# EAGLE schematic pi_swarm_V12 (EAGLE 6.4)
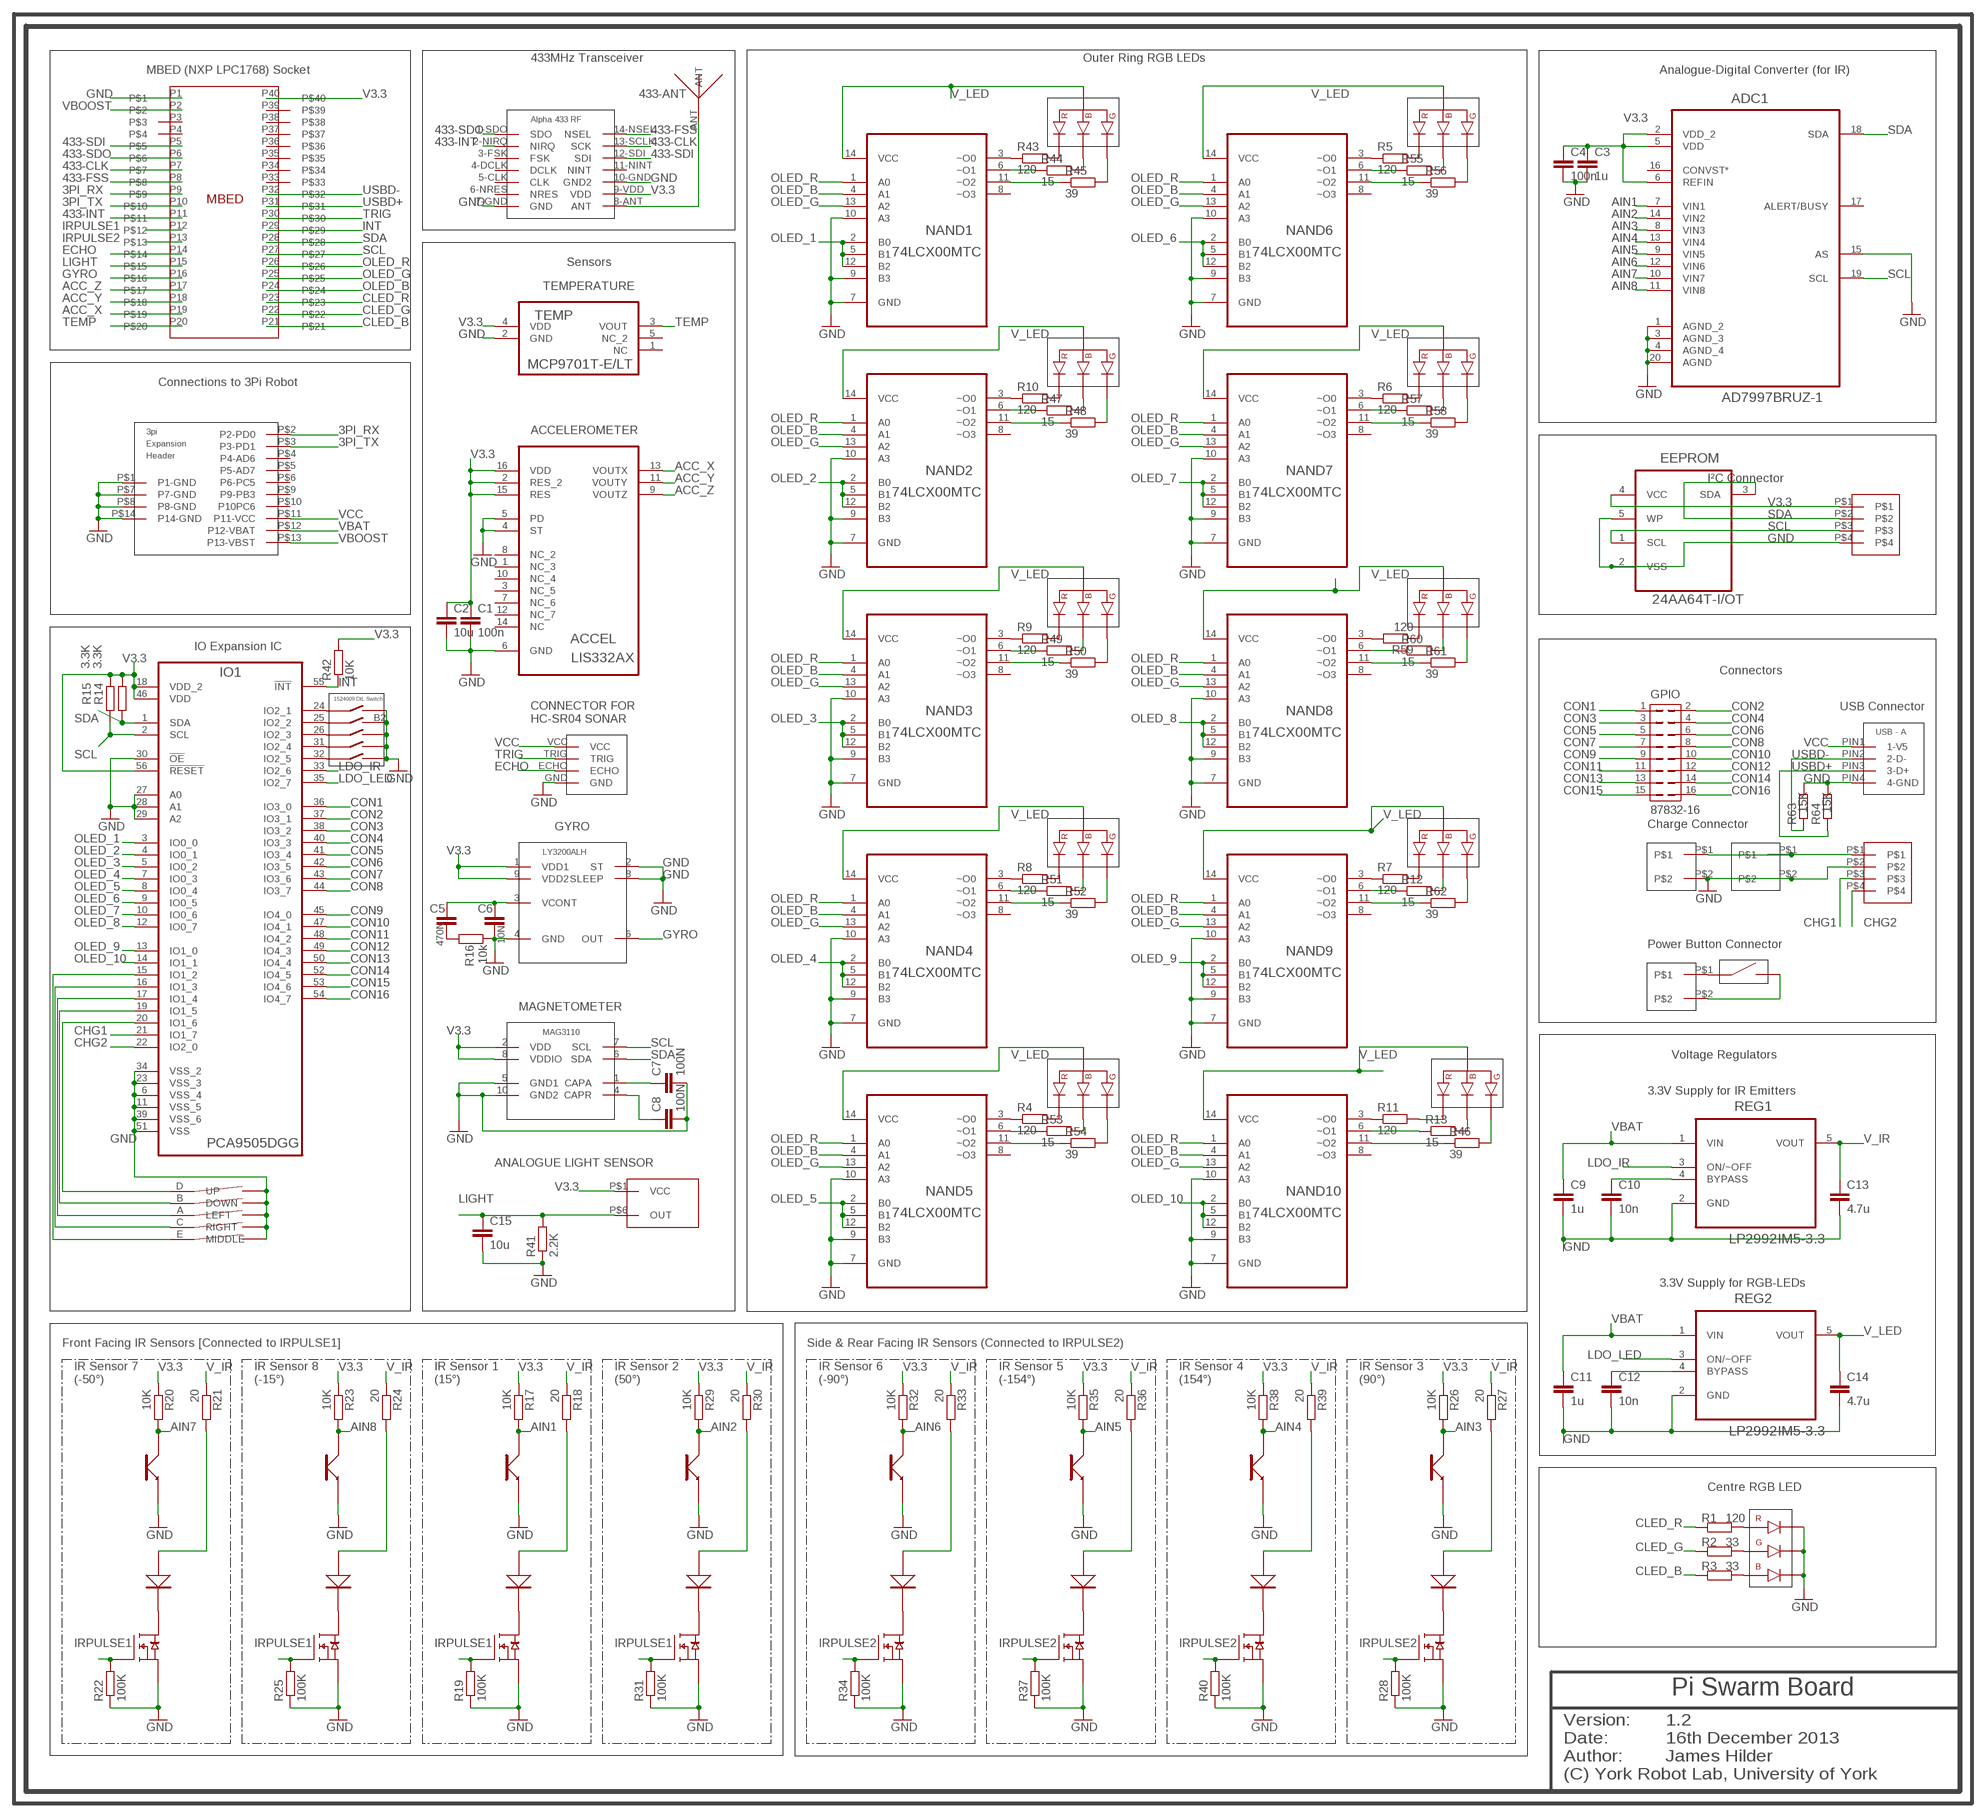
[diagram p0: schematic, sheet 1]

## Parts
3PI_HEADER  3PI-EXPANSION-HEADER  [9689605-2X7-SM-HEADER]
ACCEL  LIS332AX  [LGA16R50P3X5_300X300X100]
ADC1  AD7997BRUZ-1  [SOP65P640X120-20N]
ALPHA433  ALPHA433  [ALPHA433]
ANTENNA  ANTENNA  [2148530-433MHZANTENNA]
C1  100n  C-EUC0603  [C0603]
C2  10u  C-EUC0603  [C0603]
C3  1u  C-EUC0603  [C0603]
C4  100n  C-EUC0603  [C0603]
C5  470N  C-EUC0603  [C0603]
C6  10N  C-EUC0603  [C0603]
C7  100N  C-EUC0603  [C0603]
C8  100N  C-EUC0603  [C0603]
C9  1u  C-EUC0805K  [C0805K]
C10  10n  C-EUC0805K  [C0805K]
C11  1u  C-EUC0805K  [C0805K]
C12  10n  C-EUC0805K  [C0805K]
C13  4.7u  C-EUC1206K  [C1206K]
C14  4.7u  C-EUC1206K  [C1206K]
C15  10u  C-EUC0603K  [C0603K]
CENTRE_LED  CREE-CLP6C-FKG-RGBLED  [CREE-CLP6C-RGB-LED]
CHG_IN  2-PIN-CONNECTOR  [2-PIN-CONNECTOR]
CHG_OUT  2-PIN-CONNECTOR  [2-PIN-CONNECTOR]
EEPROM  24AA64T-I/OT  [SOT95P270X145-5N]
GPIO  87832-16  [87832-16]
GYRO  GYRO-LY3200ALH-1838547  [GYRO-1838547]
I2C_CONN  4-PIN-CONNECTOR-9492437  [4PIN-2MM-CON]
IO1  PCA9505DGG  [SOP50P810X120-56N]
IR1  TCRT1000-IR  [TCRT1000-IR]
IR2  TCRT1000-IR  [TCRT1000-IR]
IR3  TCRT1000-IR  [TCRT1000-IR]
IR4  TCRT1000-IR  [TCRT1000-IR]
IR5  TCRT1000-IR  [TCRT1000-IR]
IR6  TCRT1000-IR  [TCRT1000-IR]
IR7  TCRT1000-IR  [TCRT1000-IR]
IR8  TCRT1000-IR  [TCRT1000-IR]
LED1  KINGBRIGHT-RGL-RA-LED-2335788  [KINGBRIGHT-RA-RGB-LED]
LED2  KINGBRIGHT-RGL-RA-LED-2335788  [KINGBRIGHT-RA-RGB-LED]
LED3  KINGBRIGHT-RGL-RA-LED-2335788  [KINGBRIGHT-RA-RGB-LED]
LED4  KINGBRIGHT-RGL-RA-LED-2335788  [KINGBRIGHT-RA-RGB-LED]
LED5  KINGBRIGHT-RGL-RA-LED-2335788  [KINGBRIGHT-RA-RGB-LED]
LED6  KINGBRIGHT-RGL-RA-LED-2335788  [KINGBRIGHT-RA-RGB-LED]
LED7  KINGBRIGHT-RGL-RA-LED-2335788  [KINGBRIGHT-RA-RGB-LED]
LED8  KINGBRIGHT-RGL-RA-LED-2335788  [KINGBRIGHT-RA-RGB-LED]
LED9  KINGBRIGHT-RGL-RA-LED-2335788  [KINGBRIGHT-RA-RGB-LED]
LED10  KINGBRIGHT-RGL-RA-LED-2335788  [KINGBRIGHT-RA-RGB-LED]
LIGHTSENSOR  APDS-9005-020LIGHTSENSOR-1548110  [APDS-9005-020-LIGHTSENSOR-1548110]
MAGNETO  MAG3310-MAGNETOMETER-2080492  [MAG3110]
MBED  MBED  [MBED40PINDIL]
N1  IRLML2402-NMOS  [SOT23]
N2  IRLML2402-NMOS  [SOT23]
N3  IRLML2402-NMOS  [SOT23]
N4  IRLML2402-NMOS  [SOT23]
N5  IRLML2402-NMOS  [SOT23]
N6  IRLML2402-NMOS  [SOT23]
N7  IRLML2402-NMOS  [SOT23]
N8  IRLML2402-NMOS  [SOT23]
NAND1  74LCX00MTC  [SOP65P640X120-14N]
NAND2  74LCX00MTC  [SOP65P640X120-14N]
NAND3  74LCX00MTC  [SOP65P640X120-14N]
NAND4  74LCX00MTC  [SOP65P640X120-14N]
NAND5  74LCX00MTC  [SOP65P640X120-14N]
NAND6  74LCX00MTC  [SOP65P640X120-14N]
NAND7  74LCX00MTC  [SOP65P640X120-14N]
NAND8  74LCX00MTC  [SOP65P640X120-14N]
NAND9  74LCX00MTC  [SOP65P640X120-14N]
NAND10  74LCX00MTC  [SOP65P640X120-14N]
POWER_CON  2-PIN-CONNECTOR  [2-PIN-CONNECTOR]
R1  120  R-EU_R0603  [R0603]
R2  33  R-EU_R0603  [R0603]
R3  33  R-EU_R0603  [R0603]
R4  120  R-EU_R0603  [R0603]
R5  120  R-EU_R0603  [R0603]
R6  120  R-EU_R0603  [R0603]
R7  120  R-EU_R0603  [R0603]
R8  120  R-EU_R0603  [R0603]
R9  120  R-EU_R0603  [R0603]
R10  120  R-EU_R0603  [R0603]
R11  120  R-EU_R0603  [R0603]
R12  15  R-EU_R0603  [R0603]
R13  15  R-EU_R0603  [R0603]
R14  3.3K  R-EU_R0603  [R0603]
R15  3.3K  R-EU_R0603  [R0603]
R16  10k  R-EU_R0603  [R0603]
R17  10K  R-EU_R0603  [R0603]
R18  20  R-EU_R0603  [R0603]
R19  100K  R-EU_R0603  [R0603]
R20  10K  R-EU_R0603  [R0603]
R21  20  R-EU_R0603  [R0603]
R22  100K  R-EU_R0603  [R0603]
R23  10K  R-EU_R0603  [R0603]
R24  20  R-EU_R0603  [R0603]
R25  100K  R-EU_R0603  [R0603]
R26  10K  R-EU_R0603  [R0603]
R27  20  R-EU_R0603  [R0603]
R28  100K  R-EU_R0603  [R0603]
R29  10K  R-EU_R0603  [R0603]
R30  20  R-EU_R0603  [R0603]
R31  100K  R-EU_R0603  [R0603]
R32  10K  R-EU_R0603  [R0603]
R33  20  R-EU_R0603  [R0603]
R34  100K  R-EU_R0603  [R0603]
R35  10K  R-EU_R0603  [R0603]
R36  20  R-EU_R0603  [R0603]
R37  100K  R-EU_R0603  [R0603]
R38  10K  R-EU_R0603  [R0603]
R39  20  R-EU_R0603  [R0603]
R40  100K  R-EU_R0603  [R0603]
R41  2.2K  R-EU_R0603  [R0603]
R42  10K  R-EU_R0603  [R0603]
R43  120  R-EU_R0603  [R0603]
R44  15  R-EU_R0603  [R0603]
R45  39  R-EU_R0603  [R0603]
R46  39  R-EU_R0603  [R0603]
R47  15  R-EU_R0603  [R0603]
R48  39  R-EU_R0603  [R0603]
R49  15  R-EU_R0603  [R0603]
R50  39  R-EU_R0603  [R0603]
R51  15  R-EU_R0603  [R0603]
R52  39  R-EU_R0603  [R0603]
R53  15  R-EU_R0603  [R0603]
R54  39  R-EU_R0603  [R0603]
R55  15  R-EU_R0603  [R0603]
R56  39  R-EU_R0603  [R0603]
R57  15  R-EU_R0603  [R0603]
R58  39  R-EU_R0603  [R0603]
R59  120  R-EU_R0603  [R0603]
R60  15  R-EU_R0603  [R0603]
R61  39  R-EU_R0603  [R0603]
R62  39  R-EU_R0603  [R0603]
R63  15K  R-EU_R0402  [R0402]
R64  15K  R-EU_R0402  [R0402]
REG1  LP2992IM5-3.3  [SOT95P284X122-5N]
REG2  LP2992IM5-3.3  [SOT95P284X122-5N]
SONAR_CON  4-PIN-CONNECTOR-2084263  [4-PIN-CONNECTOR-2084263]
SWITCH1  1703878-SWITCH  [SWITCH-1703878]
SWITCH2  5WAYSWITCH-MCTT5V-1316988  [5WAYSWITCH]
SWITCH3  5PINDIPSWITCH-1524009  [5DIPSWITCH-1524009]
TEMP  MCP9701T-E/LT  [SOT65P210X110-5N]
U$1  4PIN-CON-177295  [4-PIN-CONNECTOR-1772951]
USB_CONNECTOR  USB-1654064  [USB-A-1654064]

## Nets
3PI_RX: 3PI_HEADER.P$2(P2-PD0) MBED.P9
3PI_TX: 3PI_HEADER.P$3(P3-PD1) MBED.P10
433-ANT: ALPHA433.8-ANT(ANT) ANTENNA.ANT
433-CLK: ALPHA433.13-SCLK(SCK) MBED.P7
433-FSS: ALPHA433.14-NSEL(NSEL) MBED.P8
433-INT: ALPHA433.2-NIRQ(NIRQ) MBED.P11
433-SDI: ALPHA433.12-SDI(SDI) MBED.P5
433-SDO: ALPHA433.1-SDO(SDO) MBED.P6
ACC_X: ACCEL.13(VOUTX) MBED.P19
ACC_Y: ACCEL.11(VOUTY) MBED.P18
ACC_Z: ACCEL.9(VOUTZ) MBED.P17
AIN1: ADC1.7(VIN1) IR1.4-COLLECTOR(CO) R17.2
AIN2: ADC1.14(VIN2) IR2.4-COLLECTOR(CO) R29.2
AIN3: ADC1.8(VIN3) IR3.4-COLLECTOR(CO) R26.2
AIN4: ADC1.13(VIN4) IR4.4-COLLECTOR(CO) R38.2
AIN5: ADC1.9(VIN5) IR5.4-COLLECTOR(CO) R35.2
AIN6: ADC1.12(VIN6) IR6.4-COLLECTOR(CO) R32.2
AIN7: ADC1.10(VIN7) IR7.4-COLLECTOR(CO) R20.2
AIN8: ADC1.11(VIN8) IR8.4-COLLECTOR(CO) R23.2
CHG1: IO1.21(IO1_7) U$1.P$3
CHG2: IO1.22(IO2_0) U$1.P$4
CLED_B: MBED.P21 R3.1
CLED_G: MBED.P22 R2.1
CLED_R: MBED.P23 R1.1
CON1: GPIO.1 IO1.36(IO3_0)
CON2: GPIO.2 IO1.37(IO3_1)
CON3: GPIO.3 IO1.38(IO3_2)
CON4: GPIO.4 IO1.40(IO3_3)
CON5: GPIO.5 IO1.41(IO3_4)
CON6: GPIO.6 IO1.42(IO3_5)
CON7: GPIO.7 IO1.43(IO3_6)
CON8: GPIO.8 IO1.44(IO3_7)
CON9: GPIO.9 IO1.45(IO4_0)
CON10: GPIO.10 IO1.47(IO4_1)
CON11: GPIO.11 IO1.48(IO4_2)
CON12: GPIO.12 IO1.49(IO4_3)
CON13: GPIO.13 IO1.50(IO4_4)
CON14: GPIO.14 IO1.52(IO4_5)
CON15: GPIO.15 IO1.53(IO4_6)
CON16: GPIO.16 IO1.54(IO4_7)
ECHO: MBED.P14 SONAR_CON.ECHO
GND: 3PI_HEADER.P$1(P1-GND) 3PI_HEADER.P$7(P7-GND) 3PI_HEADER.P$8(P8-GND) 3PI_HEADER.P$14(P14-GND) ACCEL.4(ST) ACCEL.5(PD) ACCEL.6(GND) ADC1.1(AGND_2) ADC1.3(AGND_3) ADC1.4(AGND_4) ADC1.15(AS) ADC1.20(AGND) ALPHA433.7-GND(GND) ALPHA433.10-GND(GND2) C1.2 C2.2 C3.2 C4.2 C6.2 C7.2 C8.2 C9.2 C10.2 C11.2 C12.2 C13.2 C14.2 C15.2 CENTRE_LED.P$4 CENTRE_LED.P$5 CENTRE_LED.P$6 CHG_IN.P$2 CHG_OUT.P$2 EEPROM.2(VSS) EEPROM.5(WP) GYRO.2(ST) GYRO.4(GND) GYRO.8(SLEEP) I2C_CONN.P$4 IO1.6(VSS_4) IO1.11(VSS_5) IO1.23(VSS_3) IO1.27(A0) IO1.28(A1) IO1.29(A2) IO1.30(!OE) IO1.34(VSS_2) IO1.39(VSS_6) IO1.51(VSS) IR1.3-EMITTER(EM) IR2.3-EMITTER(EM) IR3.3-EMITTER(EM) IR4.3-EMITTER(EM) IR5.3-EMITTER(EM) IR6.3-EMITTER(EM) IR7.3-EMITTER(EM) IR8.3-EMITTER(EM) MAGNETO.5(GND1) MAGNETO.10(GND2) MBED.P1 N1.2(2:S) N2.2(2:S) N3.2(2:S) N4.2(2:S) N5.2(2:S) N6.2(2:S) N7.2(2:S) N8.2(2:S) NAND1.7(GND) NAND1.9(B3) NAND1.10(A3) NAND2.7(GND) NAND2.9(B3) NAND2.10(A3) NAND3.7(GND) NAND3.9(B3) NAND3.10(A3) NAND4.7(GND) NAND4.9(B3) NAND4.10(A3) NAND5.7(GND) NAND5.9(B3) NAND5.10(A3) NAND6.7(GND) NAND6.9(B3) NAND6.10(A3) NAND7.7(GND) NAND7.9(B3) NAND7.10(A3) NAND8.7(GND) NAND8.9(B3) NAND8.10(A3) NAND9.7(GND) NAND9.9(B3) NAND9.10(A3) NAND10.7(GND) NAND10.9(B3) NAND10.10(A3) R16.1 R19.1 R22.1 R25.1 R28.1 R31.1 R34.1 R37.1 R40.1 R41.1 R63.2 R64.2 REG1.2(GND) REG2.2(GND) SONAR_CON.GND SWITCH2.COM1(LEFT_COMMON) SWITCH2.COM2(DOWN_COMMON) SWITCH2.COM3(UP_COMMON) SWITCH2.COM4(RIGHT_COMMON) SWITCH2.COM5(MIDDLE_COMMON) SWITCH3.A2 SWITCH3.B2 SWITCH3.C2 SWITCH3.D2 SWITCH3.E2 TEMP.2(GND) U$1.P$2 USB_CONNECTOR.PIN4(4-GND)
GYRO: GYRO.6(OUT) MBED.P16
INT: IO1.55(!INT) MBED.P29 R42.1
IRPULSE1: MBED.P12 N1.1(1:G) N2.1(1:G) N7.1(1:G) N8.1(1:G) R19.2 R22.2 R25.2 R31.2
IRPULSE2: MBED.P13 N3.1(1:G) N4.1(1:G) N5.1(1:G) N6.1(1:G) R28.2 R34.2 R37.2 R40.2
LDO_IR: IO1.33(IO2_6) REG1.3(ON/~OFF)
LDO_LED: IO1.35(IO2_7) REG2.3(ON/~OFF)
LIGHT: C15.1 LIGHTSENSOR.P$6(OUT) MBED.P15 R41.2
N$1: CENTRE_LED.P$1 R1.2
N$2: CENTRE_LED.P$2 R2.2
N$3: CENTRE_LED.P$3 R3.2
N$4: POWER_CON.P$1 SWITCH1.1
N$5: POWER_CON.P$2 SWITCH1.2
N$6: LED5.PIN1(RED_CATHODE) R4.2
N$7: LED6.PIN1(RED_CATHODE) R5.2
N$8: LED7.PIN1(RED_CATHODE) R6.2
N$9: NAND9.3(~O0) R7.1
N$10: LED4.PIN1(RED_CATHODE) R8.2
N$11: LED3.PIN1(RED_CATHODE) R9.2
N$12: LED2.PIN1(RED_CATHODE) R10.2
N$13: NAND10.3(~O0) R11.1
N$14: LED9.PIN4(BLUE_CATHODE) R12.2
N$15: LED10.PIN1(RED_CATHODE) R11.2
N$16: LED1.PIN1(RED_CATHODE) R43.2
N$17: NAND1.6(~O1) R44.1
N$18: LED1.PIN4(BLUE_CATHODE) R44.2
N$19: NAND2.3(~O0) R10.1
N$20: LED2.PIN4(BLUE_CATHODE) R47.2
N$21: LED2.PIN3(GREEN_CATHODE) R48.2
N$22: NAND3.3(~O0) R9.1
N$23: NAND3.6(~O1) R49.1
N$24: LED3.PIN4(BLUE_CATHODE) R49.2
N$25: NAND4.3(~O0) R8.1
N$26: NAND4.6(~O1) R51.1
N$27: NAND4.11(~O2) R52.1
N$28: NAND5.3(~O0) R4.1
N$29: NAND5.6(~O1) R53.1
N$30: NAND5.11(~O2) R54.1
N$31: NAND6.3(~O0) R5.1
N$32: NAND6.6(~O1) R55.1
N$33: NAND6.11(~O2) R56.1
N$34: NAND7.3(~O0) R6.1
N$35: LED7.PIN4(BLUE_CATHODE) R57.2
N$36: LED7.PIN3(GREEN_CATHODE) R58.2
N$37: NAND8.3(~O0) R59.2
N$38: NAND8.6(~O1) R60.1
N$39: LED8.PIN3(GREEN_CATHODE) R61.2
N$40: LED9.PIN1(RED_CATHODE) R7.2
N$41: NAND9.6(~O1) R12.1
N$42: NAND9.11(~O2) R62.1
N$43: LED10.PIN4(BLUE_CATHODE) R13.2
N$44: NAND10.6(~O1) R13.1
N$45: NAND10.11(~O2) R46.1
N$46: CHG_IN.P$1 CHG_OUT.P$1 U$1.P$1
N$47: C5.2 R16.2
N$48: C7.1 MAGNETO.1(CAPA)
N$49: C5.1 C6.1 GYRO.3(VCONT)
N$50: C8.1 MAGNETO.4(CAPR)
N$51: IR1.2-CATHODE(CA) N1.3(3:D)
N$52: C12.1 REG2.4(BYPASS)
N$53: C10.1 REG1.4(BYPASS)
N$54: IR7.2-CATHODE(CA) N7.3(3:D)
N$55: IR7.1-ANODE(AN) R21.2
N$56: IR1.1-ANODE(AN) R18.2
N$57: IR8.1-ANODE(AN) R24.2
N$58: IR8.2-CATHODE(CA) N8.3(3:D)
N$59: IR3.1-ANODE(AN) R27.2
N$60: IR3.2-CATHODE(CA) N3.3(3:D)
N$61: IR2.1-ANODE(AN) R30.2
N$62: IO1.15(IO1_2) SWITCH2.E(MIDDLE)
N$63: IO1.16(IO1_3) SWITCH2.C(RIGHT)
N$64: IO1.17(IO1_4) SWITCH2.A(LEFT)
N$65: IO1.19(IO1_5) SWITCH2.B(DOWN)
N$66: IO1.20(IO1_6) SWITCH2.D(UP)
N$67: IO1.24(IO2_1) SWITCH3.A1
N$68: IO1.25(IO2_2) SWITCH3.B1
N$69: IO1.26(IO2_3) SWITCH3.C1
N$70: IO1.31(IO2_4) SWITCH3.D1
N$71: IO1.32(IO2_5) SWITCH3.E1
N$72: IR6.1-ANODE(AN) R33.2
N$73: IR2.2-CATHODE(CA) N2.3(3:D)
N$74: IR5.1-ANODE(AN) R36.2
N$75: IR6.2-CATHODE(CA) N6.3(3:D)
N$76: IR5.2-CATHODE(CA) N5.3(3:D)
N$77: IR4.1-ANODE(AN) R39.2
N$78: IR4.2-CATHODE(CA) N4.3(3:D)
N$79: NAND1.3(~O0) R43.1
N$80: LED1.PIN3(GREEN_CATHODE) R45.2
N$81: NAND1.11(~O2) R45.1
N$82: LED10.PIN3(GREEN_CATHODE) R46.2
N$83: NAND2.6(~O1) R47.1
N$84: NAND2.11(~O2) R48.1
N$85: LED3.PIN3(GREEN_CATHODE) R50.2
N$86: NAND3.11(~O2) R50.1
N$87: LED4.PIN3(GREEN_CATHODE) R52.2
N$88: LED4.PIN4(BLUE_CATHODE) R51.2
N$89: LED5.PIN3(GREEN_CATHODE) R54.2
N$90: LED5.PIN4(BLUE_CATHODE) R53.2
N$91: LED6.PIN4(BLUE_CATHODE) R55.2
N$92: LED6.PIN3(GREEN_CATHODE) R56.2
N$93: NAND7.6(~O1) R57.1
N$94: NAND7.11(~O2) R58.1
N$95: LED8.PIN1(RED_CATHODE) R59.1
N$96: LED8.PIN4(BLUE_CATHODE) R60.2
N$97: NAND8.11(~O2) R61.1
N$98: LED9.PIN3(GREEN_CATHODE) R62.2
OLED_1: IO1.3(IO0_0) NAND1.2(B0) NAND1.5(B1) NAND1.12(B2)
OLED_2: IO1.4(IO0_1) NAND2.2(B0) NAND2.5(B1) NAND2.12(B2)
OLED_3: IO1.5(IO0_2) NAND3.2(B0) NAND3.5(B1) NAND3.12(B2)
OLED_4: IO1.7(IO0_3) NAND4.2(B0) NAND4.5(B1) NAND4.12(B2)
OLED_5: IO1.8(IO0_4) NAND5.2(B0) NAND5.5(B1) NAND5.12(B2)
OLED_6: IO1.9(IO0_5) NAND6.2(B0) NAND6.5(B1) NAND6.12(B2)
OLED_7: IO1.10(IO0_6) NAND7.2(B0) NAND7.5(B1) NAND7.12(B2)
OLED_8: IO1.12(IO0_7) NAND8.2(B0) NAND8.5(B1) NAND8.12(B2)
OLED_9: IO1.13(IO1_0) NAND9.2(B0) NAND9.5(B1) NAND9.12(B2)
OLED_10: IO1.14(IO1_1) NAND10.2(B0) NAND10.5(B1) NAND10.12(B2)
OLED_B: MBED.P24 NAND1.4(A1) NAND2.4(A1) NAND3.4(A1) NAND4.4(A1) NAND5.4(A1) NAND6.4(A1) NAND7.4(A1) NAND8.4(A1) NAND9.4(A1) NAND10.4(A1)
OLED_G: MBED.P25 NAND1.13(A2) NAND2.13(A2) NAND3.13(A2) NAND4.13(A2) NAND5.13(A2) NAND6.13(A2) NAND7.13(A2) NAND8.13(A2) NAND9.13(A2) NAND10.13(A2)
OLED_R: MBED.P26 NAND1.1(A0) NAND2.1(A0) NAND3.1(A0) NAND4.1(A0) NAND5.1(A0) NAND6.1(A0) NAND7.1(A0) NAND8.1(A0) NAND9.1(A0) NAND10.1(A0)
SCL: ADC1.19(SCL) EEPROM.1(SCL) I2C_CONN.P$3 IO1.2(SCL) MAGNETO.7(SCL) MBED.P27 R15.1
SDA: ADC1.18(SDA) EEPROM.3(SDA) I2C_CONN.P$2 IO1.1(SDA) MAGNETO.6(SDA) MBED.P28 R14.1
TEMP: MBED.P20 TEMP.3(VOUT)
TRIG: MBED.P30 SONAR_CON.TRIG
USBD+: MBED.P31 R64.1 USB_CONNECTOR.PIN3(3-D+)
USBD-: MBED.P32 R63.1 USB_CONNECTOR.PIN2(2-D-)
V3.3: ACCEL.2(RES_2) ACCEL.15(RES) ACCEL.16(VDD) ADC1.2(VDD_2) ADC1.5(VDD) ADC1.6(REFIN) ALPHA433.9-VDD(VDD) C1.1 C2.1 C3.1 C4.1 EEPROM.4(VCC) GYRO.1(VDD1) GYRO.9(VDD2) I2C_CONN.P$1 IO1.18(VDD_2) IO1.46(VDD) IO1.56(!RESET) LIGHTSENSOR.P$1(VCC) MAGNETO.2(VDD) MAGNETO.8(VDDIO) MBED.P40 R14.2 R15.2 R17.1 R20.1 R23.1 R26.1 R29.1 R32.1 R35.1 R38.1 R42.2 TEMP.4(VDD)
V_IR: C13.1 R18.1 R21.1 R24.1 R27.1 R30.1 R33.1 R36.1 R39.1 REG1.5(VOUT)
V_LED: C14.1 LED1.PIN2(ANODE) LED2.PIN2(ANODE) LED3.PIN2(ANODE) LED4.PIN2(ANODE) LED5.PIN2(ANODE) LED6.PIN2(ANODE) LED7.PIN2(ANODE) LED8.PIN2(ANODE) LED9.PIN2(ANODE) LED10.PIN2(ANODE) NAND1.14(VCC) NAND2.14(VCC) NAND3.14(VCC) NAND4.14(VCC) NAND5.14(VCC) NAND6.14(VCC) NAND7.14(VCC) NAND8.14(VCC) NAND9.14(VCC) NAND10.14(VCC) REG2.5(VOUT)
VBAT: 3PI_HEADER.P$12(P12-VBAT) C9.1 C11.1 REG1.1(VIN) REG2.1(VIN)
VBOOST: 3PI_HEADER.P$13(P13-VBST) MBED.P2
VCC: 3PI_HEADER.P$11(P11-VCC) SONAR_CON.VCC USB_CONNECTOR.PIN1(1-V5)
Unconnected: 3PI_HEADER.P$4(P4-AD6) 3PI_HEADER.P$5(P5-AD7) 3PI_HEADER.P$6(P6-PC5) 3PI_HEADER.P$9(P9-PB3) 3PI_HEADER.P$10(P10PC6) ACCEL.1(NC_3) ACCEL.3(NC_5) ACCEL.7(NC_6) ACCEL.8(NC_2) ACCEL.10(NC_4) ACCEL.12(NC_7) ACCEL.14(NC) ADC1.16(CONVST*) ADC1.17(ALERT/BUSY) ALPHA433.3-FSK(FSK) ALPHA433.4-DCLK(DCLK) ALPHA433.5-CLK(CLK) ALPHA433.6-NRES(NRES) ALPHA433.11-NINT(NINT) MBED.P3 MBED.P4 MBED.P33 MBED.P34 MBED.P35 MBED.P36 MBED.P37 MBED.P38 MBED.P39 NAND1.8(~O3) NAND2.8(~O3) NAND3.8(~O3) NAND4.8(~O3) NAND5.8(~O3) NAND6.8(~O3) NAND7.8(~O3) NAND8.8(~O3) NAND9.8(~O3) NAND10.8(~O3) TEMP.1(NC) TEMP.5(NC_2)

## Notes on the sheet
- 433MHz Transceiver | Outer Ring RGB LEDs
- MBED (NXP LPC1768) Socket | Analogue-Digital Converter (for IR)
- Sensors
- TEMPERATURE
- Connections to 3Pi Robot
- ACCELEROMETER
- I²C Connector
- IO Expansion IC
- Connectors
- USB Connector
- CONNECTOR FOR
  HC-SR04 SONAR
- GYRO | Charge Connector
- Power Button Connector
- MAGNETOMETER
- Voltage Regulators
- 3.3V Supply for IR Emitters
- ANALOGUE LIGHT SENSOR
- 3.3V Supply for RGB-LEDs
- Front Facing IR Sensors [Connected to IRPULSE1] | Side & Rear Facing IR Sensors (Connected to IRPULSE2)
- IR Sensor 7
  (-50°)
- IR Sensor 8
  (-15°)
- IR Sensor 1
  (15°)
- IR Sensor 2
  (50°)
- IR Sensor 6
  (-90°)
- IR Sensor 5
  (-154°)
- IR Sensor 4
  (154°)
- IR Sensor 3
  (90°)
- Centre RGB LED
- Pi Swarm Board
- 1.2
  16th December 2013
  James Hilder
- Version:
  Date:
  Author:
  (C) York Robot Lab, University of York

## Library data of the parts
3PI_HEADER = pololu_library:3PI-EXPANSION-HEADER
ACCEL = pololu_library:LIS332AX: MEMS motion sensor; MPN: LIS332AX; OC_FARNELL: 1838527; OC_NEWARK: 71R6453; PACKAGE: LGA-16; SUPPLIER: STMicroelectronics
ADC1 = pololu_library:AD7997BRUZ-1: 10BIT ADC, 8CH I2C I/F, SMD; MPN: AD7997BRUZ-1; OC_FARNELL: 1078305; OC_NEWARK: 31M4429; PACKAGE: TSSOP-20; SUPPLIER: Analog Devices
ALPHA433 = pololu_library:ALPHA433
ANTENNA = pololu_library:ANTENNA
C1 C2 C5-C15 = rcl:C-EU: CAPACITOR, European symbol
C3 C4 = resistor:C-EU: CAPACITOR, European symbol
CENTRE_LED = pololu_library:CREE-CLP6C-FKG-RGBLED
CHG_IN CHG_OUT POWER_CON = pololu_library:2-PIN-CONNECTOR
EEPROM = pololu_library:24AA64T-I/OT: 64K I2C Serial EEPROM ,SOT23-5; MPN: 24AA64T-I/OT; OC_FARNELL: 2101260; OC_NEWARK: 08P0062; PACKAGE: SOT23-5; SUPPLIER: MICROCHIP
GPIO = con-molex:87832-16: Milli-Grid Header 2.00mm (.079") Pitch; OC_FARNELL: 1756949; OC_NEWARK: unknown
GYRO = pololu_library:GYRO-LY3200ALH-1838547
I2C_CONN = pololu_library:4-PIN-CONNECTOR-9492437
IO1 = pololu_library:PCA9505DGG: 40-bit I2C-bus I/O port,TSSOP-56; MPN: PCA9505DGG; OC_FARNELL: 2212087; OC_NEWARK: 55W4300; PACKAGE: TSSOP-56; SUPPLIER: NXP
IR1-IR8 = pololu_library:TCRT1000-IR
LED1-LED10 = pololu_library:KINGBRIGHT-RGL-RA-LED-2335788
LIGHTSENSOR = pololu_library:APDS-9005-020LIGHTSENSOR-1548110
MAGNETO = pololu_library:MAG3310-MAGNETOMETER-2080492
MBED = mbed:MBED
N1-N8 = pololu_library:IRLML2402-NMOS
NAND1-NAND10 = pololu_library:74LCX00MTC: Low Voltage Quad 2-Input NAND Gate with 5V Tolerant Inputs; MPN: 74LCX00MTC; OC_FARNELL: 1607738; OC_NEWARK: 78K6272; PACKAGE: TSSOP-14; SUPPLIER: FAIRCHILD
R1-R3 R11 R13-R15 R17-R46 R63 R64 = rcl:R-EU_: RESISTOR, European symbol
R4-R10 R12 R16 R47-R62 = resistor:R-EU_: RESISTOR, European symbol
REG1 REG2 = pololu_library:LP2992IM5-3.3: Low-Dropout Regulator; MPN: LP2992IM5-3.3; OC_FARNELL: 1469141; OC_NEWARK: 41K7301; PACKAGE: SOT23-5; SUPPLIER: National Semiconductor
SONAR_CON = pololu_library:4-PIN-CONNECTOR-2084263
SWITCH1 = pololu_library:1703878-SWITCH
SWITCH2 = pololu_library:5WAYSWITCH-MCTT5V-1316988
SWITCH3 = pololu_library:5PINDIPSWITCH-1524009
TEMP = pololu_library:MCP9701T-E/LT: IC, TEMPERATURE SENSOR, ± 2°C; MPN: MCP9701T-E/LT; OC_FARNELL: 1084622; OC_NEWARK: 08J8799; PACKAGE: SC70-5; SUPPLIER: Microchip
U$1 = pololu_library:4PIN-CON-177295
USB_CONNECTOR = pololu_library:USB-1654064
